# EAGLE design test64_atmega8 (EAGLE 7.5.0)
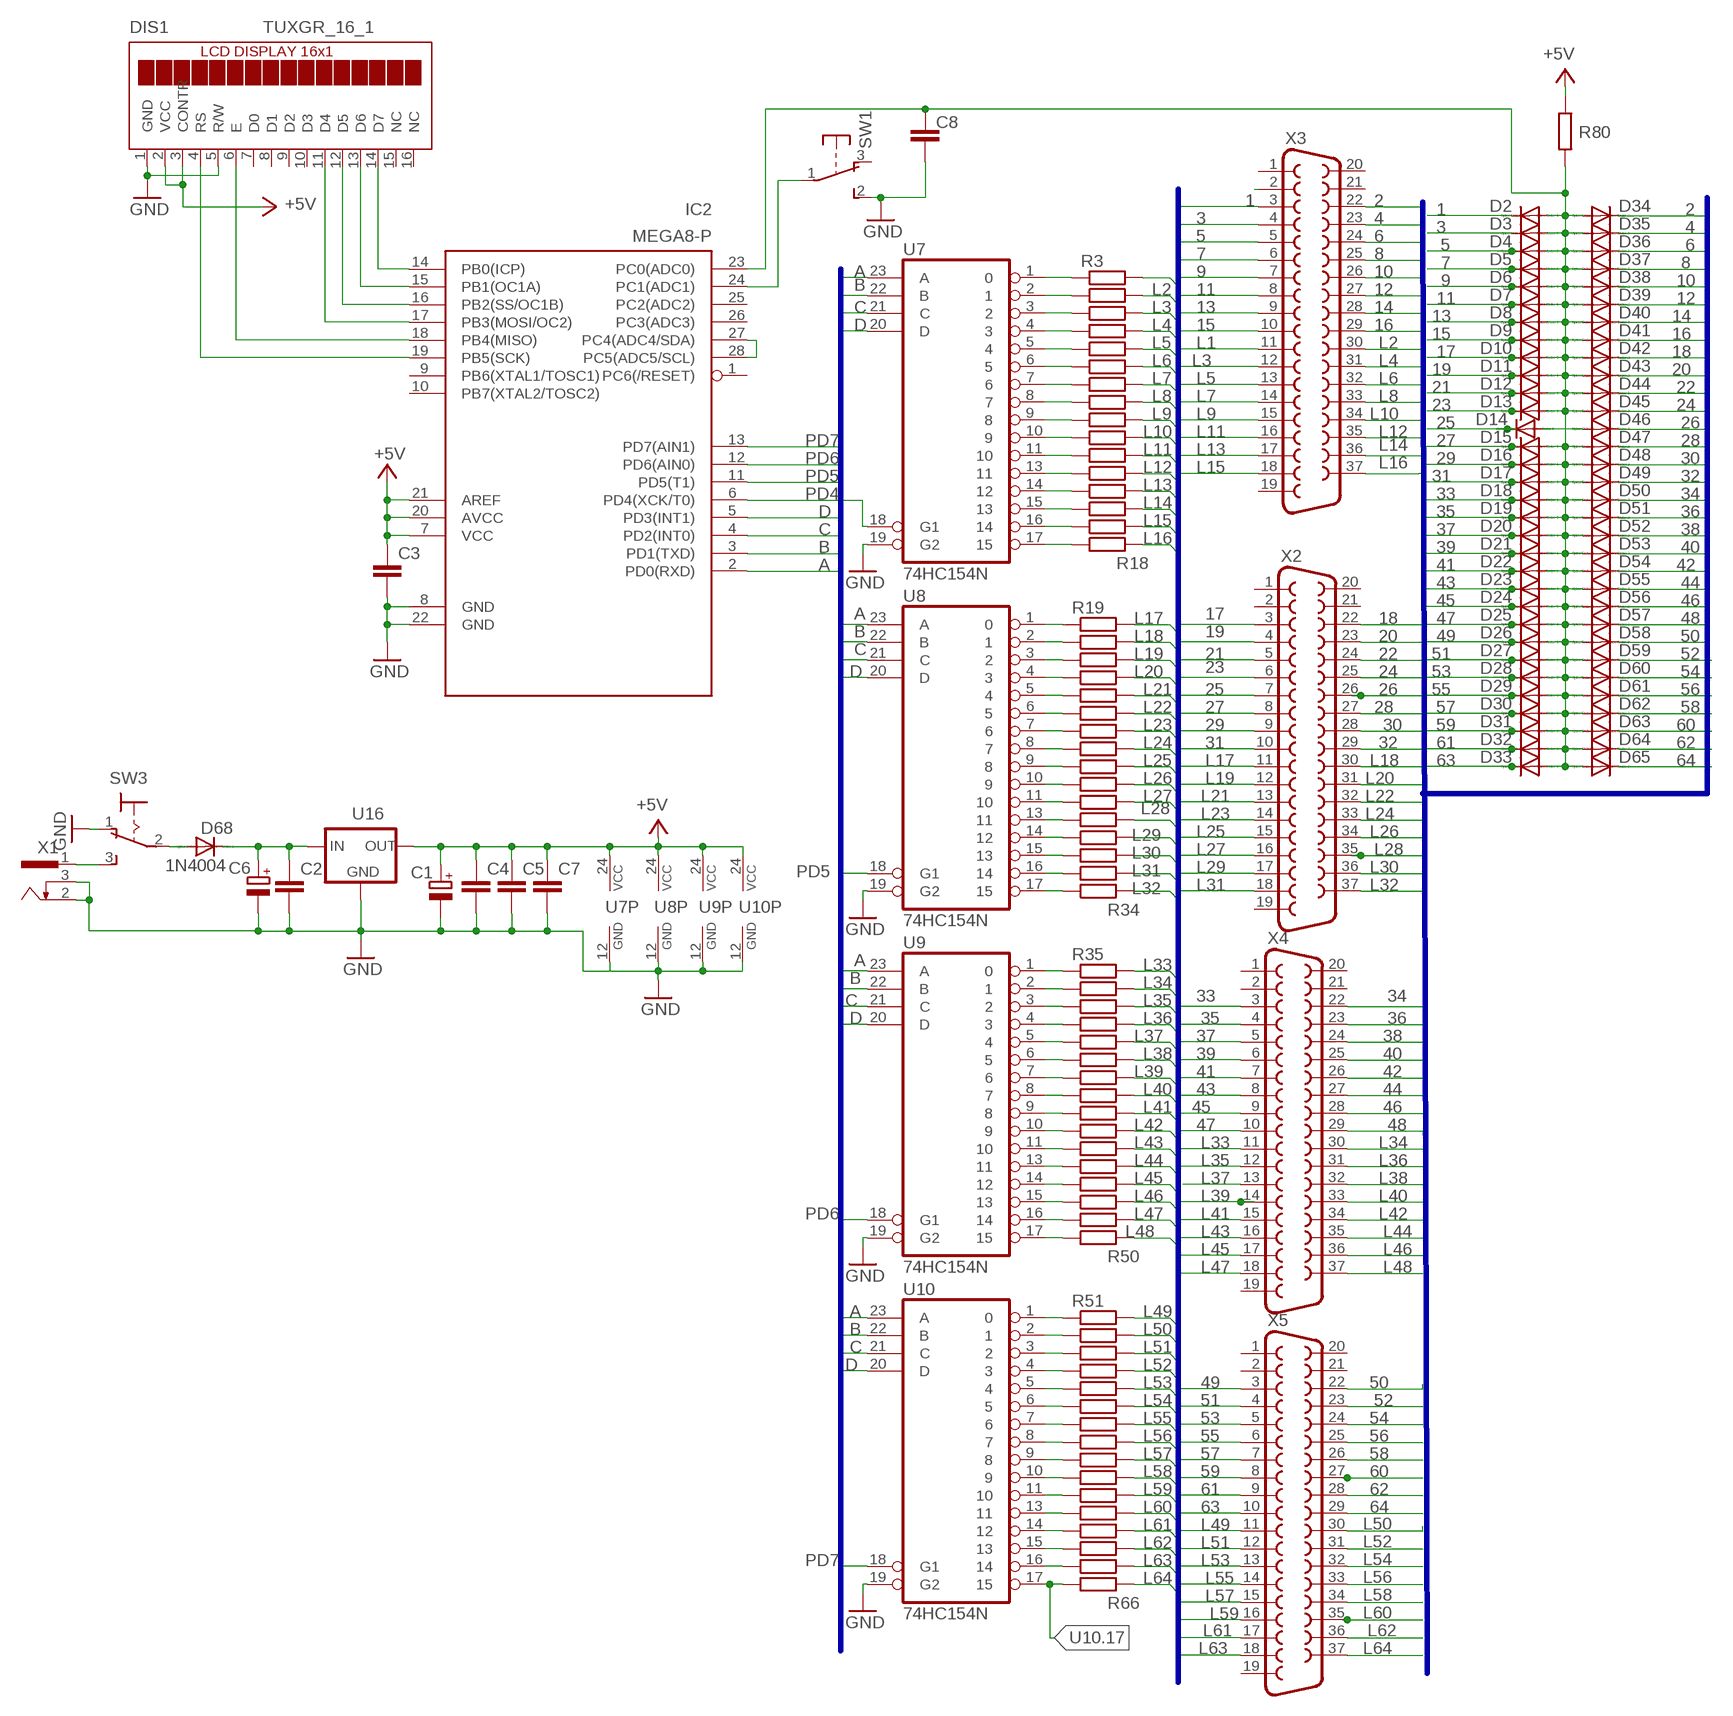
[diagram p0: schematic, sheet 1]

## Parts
C1  CPOL-EUC/6032-28W  [C/6032-28W]
C2  C-EUC1206  [C1206]
C3  C-EUC1206  [C1206]
C4  C-EUC1206  [C1206]
C5  C-EUC1206  [C1206]
C6  CPOL-EUC/6032-28W  [C/6032-28W]
C7  C-EUC1206  [C1206]
C8  C-EUC1206  [C1206]
D2  1N4148DO35-7  [DO35-7]
D3  1N4148DO35-7  [DO35-7]
D4  1N4148DO35-7  [DO35-7]
D5  1N4148DO35-7  [DO35-7]
D6  1N4148DO35-7  [DO35-7]
D7  1N4148DO35-7  [DO35-7]
D8  1N4148DO35-7  [DO35-7]
D9  1N4148DO35-7  [DO35-7]
D10  1N4148DO35-7  [DO35-7]
D11  1N4148DO35-7  [DO35-7]
D12  1N4148DO35-7  [DO35-7]
D13  1N4148DO35-7  [DO35-7]
D14  1N4148DO35-7  [DO35-7]
D15  1N4148DO35-7  [DO35-7]
D16  1N4148DO35-7  [DO35-7]
D17  1N4148DO35-7  [DO35-7]
D18  1N4148DO35-7  [DO35-7]
D19  1N4148DO35-7  [DO35-7]
D20  1N4148DO35-7  [DO35-7]
D21  1N4148DO35-7  [DO35-7]
D22  1N4148DO35-7  [DO35-7]
D23  1N4148DO35-7  [DO35-7]
D24  1N4148DO35-7  [DO35-7]
D25  1N4148DO35-7  [DO35-7]
D26  1N4148DO35-7  [DO35-7]
D27  1N4148DO35-7  [DO35-7]
D28  1N4148DO35-7  [DO35-7]
D29  1N4148DO35-7  [DO35-7]
D30  1N4148DO35-7  [DO35-7]
D31  1N4148DO35-7  [DO35-7]
D32  1N4148DO35-7  [DO35-7]
D33  1N4148DO35-7  [DO35-7]
D34  1N4148DO35-7  [DO35-7]
D35  1N4148DO35-7  [DO35-7]
D36  1N4148DO35-7  [DO35-7]
D37  1N4148DO35-7  [DO35-7]
D38  1N4148DO35-7  [DO35-7]
D39  1N4148DO35-7  [DO35-7]
D40  1N4148DO35-7  [DO35-7]
D41  1N4148DO35-7  [DO35-7]
D42  1N4148DO35-7  [DO35-7]
D43  1N4148DO35-7  [DO35-7]
D44  1N4148DO35-7  [DO35-7]
D45  1N4148DO35-7  [DO35-7]
D46  1N4148DO35-7  [DO35-7]
D47  1N4148DO35-7  [DO35-7]
D48  1N4148DO35-7  [DO35-7]
D49  1N4148DO35-7  [DO35-7]
D50  1N4148DO35-7  [DO35-7]
D51  1N4148DO35-7  [DO35-7]
D52  1N4148DO35-7  [DO35-7]
D53  1N4148DO35-7  [DO35-7]
D54  1N4148DO35-7  [DO35-7]
D55  1N4148DO35-7  [DO35-7]
D56  1N4148DO35-7  [DO35-7]
D57  1N4148DO35-7  [DO35-7]
D58  1N4148DO35-7  [DO35-7]
D59  1N4148DO35-7  [DO35-7]
D60  1N4148DO35-7  [DO35-7]
D61  1N4148DO35-7  [DO35-7]
D62  1N4148DO35-7  [DO35-7]
D63  1N4148DO35-7  [DO35-7]
D64  1N4148DO35-7  [DO35-7]
D65  1N4148DO35-7  [DO35-7]
D68  1N4004  [DO41-10]
DIS1  TUXGR_16_1  [TUXGR_16X1]
IC2  MEGA8-P  [DIL28-3]
R3  R-EU_R1206  [R1206]
R4  R-EU_R1206  [R1206]
R5  R-EU_R1206  [R1206]
R6  R-EU_R1206  [R1206]
R7  R-EU_R1206  [R1206]
R8  R-EU_R1206  [R1206]
R9  R-EU_R1206  [R1206]
R10  R-EU_R1206  [R1206]
R11  R-EU_R1206  [R1206]
R12  R-EU_R1206  [R1206]
R13  R-EU_R1206  [R1206]
R14  R-EU_R1206  [R1206]
R15  R-EU_R1206  [R1206]
R16  R-EU_R1206  [R1206]
R17  R-EU_R1206  [R1206]
R18  R-EU_R1206  [R1206]
R19  R-EU_R1206  [R1206]
R20  R-EU_R1206  [R1206]
R21  R-EU_R1206  [R1206]
R22  R-EU_R1206  [R1206]
R23  R-EU_R1206  [R1206]
R24  R-EU_R1206  [R1206]
R25  R-EU_R1206  [R1206]
R26  R-EU_R1206  [R1206]
R27  R-EU_R1206  [R1206]
R28  R-EU_R1206  [R1206]
R29  R-EU_R1206  [R1206]
R30  R-EU_R1206  [R1206]
R31  R-EU_R1206  [R1206]
R32  R-EU_R1206  [R1206]
R33  R-EU_R1206  [R1206]
R34  R-EU_R1206  [R1206]
R35  R-EU_R1206  [R1206]
R36  R-EU_R1206  [R1206]
R37  R-EU_R1206  [R1206]
R38  R-EU_R1206  [R1206]
R39  R-EU_R1206  [R1206]
R40  R-EU_R1206  [R1206]
R41  R-EU_R1206  [R1206]
R42  R-EU_R1206  [R1206]
R43  R-EU_R1206  [R1206]
R44  R-EU_R1206  [R1206]
R45  R-EU_R1206  [R1206]
R46  R-EU_R1206  [R1206]
R47  R-EU_R1206  [R1206]
R48  R-EU_R1206  [R1206]
R49  R-EU_R1206  [R1206]
R50  R-EU_R1206  [R1206]
R51  R-EU_R1206  [R1206]
R52  R-EU_R1206  [R1206]
R53  R-EU_R1206  [R1206]
R54  R-EU_R1206  [R1206]
R55  R-EU_R1206  [R1206]
R56  R-EU_R1206  [R1206]
R57  R-EU_R1206  [R1206]
R58  R-EU_R1206  [R1206]
R59  R-EU_R1206  [R1206]
R60  R-EU_R1206  [R1206]
R61  R-EU_R1206  [R1206]
R62  R-EU_R1206  [R1206]
R63  R-EU_R1206  [R1206]
R64  R-EU_R1206  [R1206]
R65  R-EU_R1206  [R1206]
R66  R-EU_R1206  [R1206]
R80  R-EU_R1206  [R1206]
SW1  9077-1  [9077-1]
SW3  320-916  [320-916]
U7  74HC154N  [DIL24-6]
U8  74HC154N  [DIL24-6]
U9  74HC154N  [DIL24-6]
U10  74HC154N  [DIL24-6]
U16  78XXL  [78XXL]
X1  733980-62  [733980-62]
X2  F37V  [F37V]
X3  F37V  [F37V]
X4  F37V  [F37V]
X5  F37V  [F37V]

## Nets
1: D2.C X3.3
2: D34.C X3.22
3: D3.C X3.4
4: D35.C X3.23
5: D4.C X3.5
6: D36.C X3.24
7: D5.C X3.6
8: D37.C X3.25
9: D6.C X3.7
10: D38.C X3.26
11: D7.C X3.8
12: D39.C X3.27
13: D8.C X3.9
14: D40.C X3.28
15: D9.C X3.10
16: D41.C X3.29
17: D10.C X2.3
18: D42.C X2.22
19: D11.C X2.4
20: D43.C X2.23
21: D12.C X2.5
22: D44.C X2.24
23: D13.C X2.6
24: D45.C X2.25
25: D14.C X2.7
26: D46.C X2.26
27: D15.C X2.8
28: D47.C X2.27
29: D16.C X2.9
30: D48.C X2.28
31: D17.C X2.10
32: D49.C X2.29
33: D18.C X4.3
34: D50.C X4.22
35: D19.C X4.4
36: D51.C X4.23
37: D20.C X4.5
38: D52.C X4.24
39: D21.C X4.6
40: D53.C X4.25
41: D22.C X4.7
42: D54.C X4.26
43: D23.C X4.8
44: D55.C X4.27
45: D24.C X4.9
46: D56.C X4.28
47: D25.C X4.10
48: D57.C X4.29
49: D26.C X5.3
50: D58.C X5.22
51: D27.C X5.4
52: D59.C X5.23
53: D28.C X5.5
54: D60.C X5.24
55: D29.C X5.6
56: D61.C X5.25
57: D30.C X5.7
58: D62.C X5.26
59: D31.C X5.8
60: D63.C X5.27
61: D32.C X5.9
62: D64.C X5.28
63: D33.C X5.10
64: D65.C X5.29
+5V: C1.+ C3.1 C4.1 C5.1 C7.1 DIS1.2(VCC) DIS1.3(CONTR) IC2.7(VCC) IC2.20(AVCC) IC2.21(AREF) R80.1 U7.24(VCC) U8.24(VCC) U9.24(VCC) U10.24(VCC) U16.OUT
A: IC2.2(PD0(RXD)) U7.23(A) U8.23(A) U9.23(A) U10.23(A)
B: IC2.3(PD1(TXD)) U7.22(B) U8.22(B) U9.22(B) U10.22(B)
C: IC2.4(PD2(INT0)) U7.21(C) U8.21(C) U9.21(C) U10.21(C)
D: IC2.5(PD3(INT1)) U7.20(D) U8.20(D) U9.20(D) U10.20(D)
GND: C1.- C2.2 C3.2 C4.2 C5.2 C6.- C7.2 C8.2 DIS1.1(GND) DIS1.5(R/W) IC2.8(GND) IC2.22(GND) SW1.2(S) SW3.1(O) U7.12(GND) U7.19(G2) U8.12(GND) U8.19(G2) U9.12(GND) U9.19(G2) U10.12(GND) U10.19(G2) U16.GND X1.2 X1.3
L1: R3.2 X3.11
L2: R4.2 X3.30
L3: R5.2 X3.12
L4: R6.2 X3.31
L5: R7.2 X3.13
L6: R8.2 X3.32
L7: R9.2 X3.14
L8: R10.2 X3.33
L9: R11.2 X3.15
L10: R12.2 X3.34
L11: R13.2 X3.16
L12: R14.2 X3.35
L13: R15.2 X3.17
L14: R16.2 X3.36
L15: R17.2 X3.18
L16: R18.2 X3.37
L17: R19.2 X2.11
L18: R20.2 X2.30
L19: R21.2 X2.12
L20: R22.2 X2.31
L21: R23.2 X2.13
L22: R24.2 X2.32
L23: R25.2 X2.14
L24: R26.2 X2.33
L25: R27.2 X2.15
L26: R28.2 X2.34
L27: R29.2 X2.16
L28: R30.2 X2.35
L29: R31.2 X2.17
L30: R32.2 X2.36
L31: R33.2 X2.18
L32: R34.2 X2.37
L33: R35.2 X4.11
L34: R36.2 X4.30
L35: R37.2 X4.12
L36: R38.2 X4.31
L37: R39.2 X4.13
L38: R40.2 X4.32
L39: R41.2 X4.14
L40: R42.2 X4.33
L41: R43.2 X4.15
L42: R44.2 X4.34
L43: R45.2 X4.16
L44: R46.2 X4.35
L45: R47.2 X4.17
L46: R48.2 X4.36
L47: R49.2 X4.18
L48: R50.2 X4.37
L49: R51.2 X5.11
L50: R52.2 X5.30
L51: R53.2 X5.12
L52: R54.2 X5.31
L53: R55.2 X5.13
L54: R56.2 X5.32
L55: R57.2 X5.14
L56: R58.2 X5.33
L57: R59.2 X5.15
L58: R60.2 X5.34
L59: R61.2 X5.16
L60: R62.2 X5.35
L61: R63.2 X5.17
L62: R64.2 X5.36
L63: R65.2 X5.18
L64: R66.2 X5.37
N$1: IC2.27(PC4(ADC4/SDA)) IC2.28(PC5(ADC5/SCL))
N$2: IC2.24(PC1(ADC1)) SW1.1(P)
N$3: DIS1.14(D7) IC2.14(PB0(ICP))
N$4: DIS1.13(D6) IC2.15(PB1(OC1A))
N$5: DIS1.12(D5) IC2.16(PB2(SS/OC1B))
N$6: DIS1.11(D4) IC2.17(PB3(MOSI/OC2))
N$7: R4.1 U7.2
N$8: R5.1 U7.3
N$9: R6.1 U7.4
N$10: R7.1 U7.5
N$11: R8.1 U7.6
N$12: R9.1 U7.7
N$13: R10.1 U7.8
N$14: R11.1 U7.9
N$15: R12.1 U7.10
N$16: R13.1 U7.11
N$17: R14.1 U7.13
N$18: R15.1 U7.14
N$19: R16.1 U7.15
N$20: R17.1 U7.16
N$21: R18.1 U7.17
N$22: R19.1 U8.1
N$23: R20.1 U8.2
N$24: R21.1 U8.3
N$25: R22.1 U8.4
N$26: R23.1 U8.5
N$27: R24.1 U8.6
N$28: R25.1 U8.7
N$29: R26.1 U8.8
N$30: R27.1 U8.9
N$31: R28.1 U8.10
N$32: R29.1 U8.11
N$33: R30.1 U8.13
N$34: R31.1 U8.14
N$35: R32.1 U8.15
N$36: R33.1 U8.16
N$37: R34.1 U8.17
N$38: R35.1 U9.1
N$39: R36.1 U9.2
N$40: R37.1 U9.3
N$41: R38.1 U9.4
N$42: R39.1 U9.5
N$43: R40.1 U9.6
N$44: R41.1 U9.7
N$45: R42.1 U9.8
N$46: R43.1 U9.9
N$47: R44.1 U9.10
N$48: R45.1 U9.11
N$49: R46.1 U9.13
N$50: R47.1 U9.14
N$51: R48.1 U9.15
N$52: R49.1 U9.16
N$53: R50.1 U9.17
N$54: R51.1 U10.1
N$55: R52.1 U10.2
N$56: R53.1 U10.3
N$57: R54.1 U10.4
N$58: R55.1 U10.5
N$59: R56.1 U10.6
N$60: R57.1 U10.7
N$61: R58.1 U10.8
N$62: R59.1 U10.9
N$63: R60.1 U10.10
N$64: R61.1 U10.11
N$65: R62.1 U10.13
N$66: R63.1 U10.14
N$67: R64.1 U10.15
N$68: R65.1 U10.16
N$69: DIS1.6(E) IC2.18(PB4(MISO))
N$70: DIS1.4(RS) IC2.19(PB5(SCK))
N$71: X3.2
N$72: R3.1 U7.1
N$95: D68.A SW3.2(P)
N$109: C8.1 D2.A D3.A D4.A D5.A D6.A D7.A D8.A D9.A D10.A D11.A D12.A D13.A D14.A D15.A D16.A D17.A D18.A D19.A D20.A D21.A D22.A D23.A D24.A D25.A D26.A D27.A D28.A D29.A D30.A D31.A D32.A D33.A D34.A D35.A D36.A D37.A D38.A D39.A D40.A D41.A D42.A D43.A D44.A D45.A D46.A D47.A D48.A D49.A D50.A D51.A D52.A D53.A D54.A D55.A D56.A D57.A D58.A D59.A D60.A D61.A D62.A D63.A D64.A D65.A IC2.23(PC0(ADC0)) R80.2
N$118: C2.1 C6.+ D68.C U16.IN
N$119: SW3.3(S) X1.1
PD4: IC2.6(PD4(XCK/T0)) U7.18(G1)
PD5: IC2.11(PD5(T1)) U8.18(G1)
PD6: IC2.12(PD6(AIN0)) U9.18(G1)
PD7: IC2.13(PD7(AIN1)) U10.18(G1)
U10.17: R66.1 U10.17
Unconnected: DIS1.7(D0) DIS1.8(D1) DIS1.9(D2) DIS1.10(D3) DIS1.15(NC) DIS1.16(NC) IC2.1(PC6(/RESET)) IC2.9(PB6(XTAL1/TOSC1)) IC2.10(PB7(XTAL2/TOSC2)) IC2.25(PC2(ADC2)) IC2.26(PC3(ADC3)) SW1.3(O) X2.1 X2.2 X2.19 X2.20 X2.21 X3.1 X3.19 X3.20 X3.21 X4.1 X4.2 X4.19 X4.20 X4.21 X5.1 X5.2 X5.19 X5.20 X5.21

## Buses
B$1
B$2
B$3

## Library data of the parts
C1 C6 = rcl:CPOL-EU: POLARIZED CAPACITOR, European symbol
C2-C5 C7 C8 = rcl:C-EU: CAPACITOR, European symbol
D2-D65 = diode:1N4148: DIODE
D68 = diode:1N4004: DIODE
DIS1 = display-lcd:TUXGR_16_1: 1x16 LCD DISPLAY
IC2 = atmel:MEGA8-P: MICROCONTROLLER 8 Kbytes FLASH, 1 kbytes SRAM, 512 bytes EEPROM, USART, 4-channel 10 bit ADC, 2-channel 8 bit ADC Pin compatible with Atmega48, ATMega88, ATMega168 Source: avr.lbr; OC_FARNELL: unknown; OC_NEWARK: unknown
R3-R66 R80 = rcl:R-EU_: RESISTOR, European symbol
SW1 = switch-misc:9077-1: MARQUARDT SWITCH 9077.0100 Distributor: Buerklin
SW3 = switch:320-916: TOGGLE SWITCH distributor RS Components
U7-U10 = 74xx-eu:74*154: 4-line to 16-line data SELECTOR/MULTIPLEXER
U16 = v-reg:78XXL: VOLTAGE REGULATOR
X1 = con-conrad:73398?: FEMALE PRINT CONNECTOR Niedervolt-Steckverbinder Distributor Conrad
X2-X5 = con-subd:F37: SUB-D; OC_FARNELL: unknown; OC_NEWARK: unknown

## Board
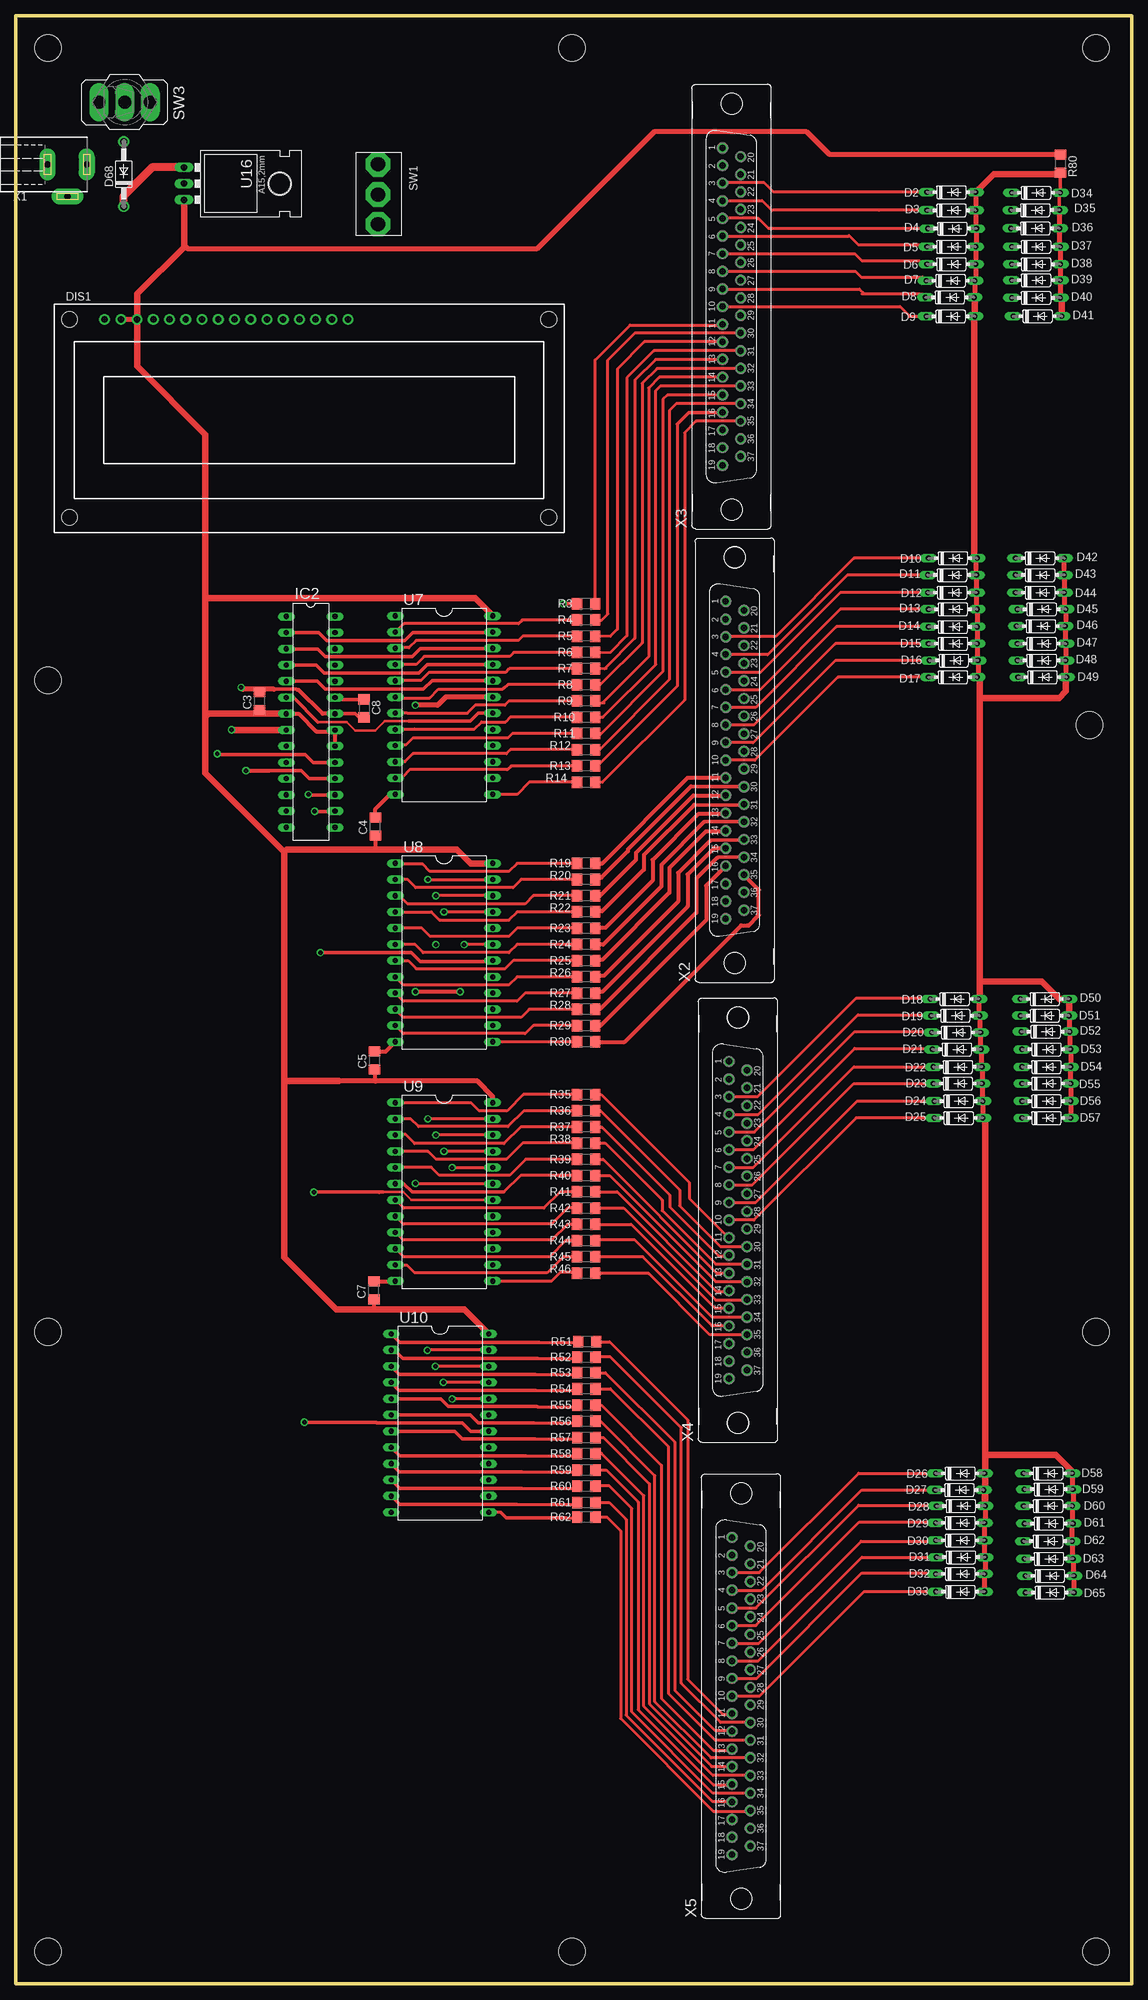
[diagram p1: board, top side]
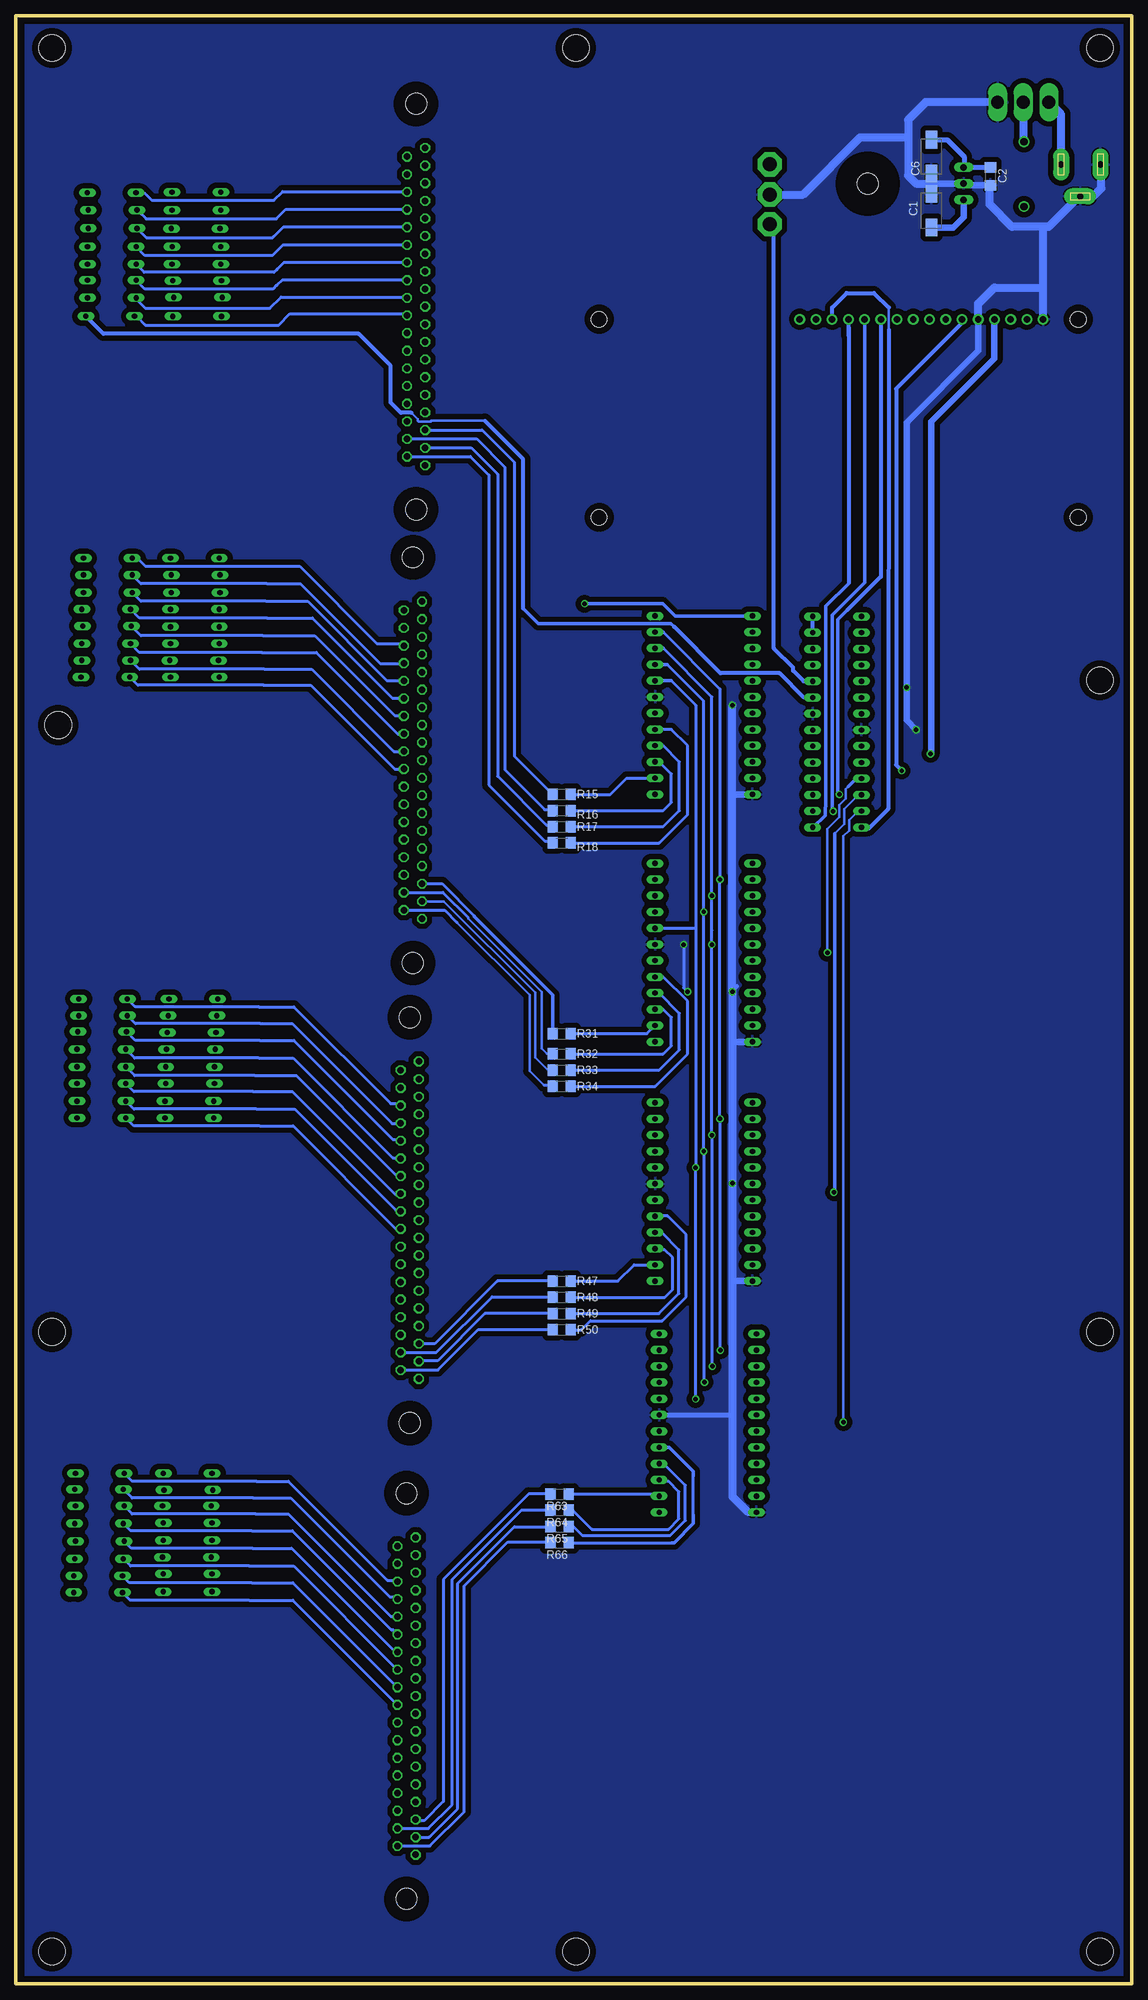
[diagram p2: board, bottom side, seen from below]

Size 174.62 x 308 mm. Coordinates in mm from the lower left corner, seen from the top.
Outline: 0,0 0,308 174.62,308 174.62,0 0,0
Copper layers (1*16): Top 0.035mm / dielectric 1.5mm / Bottom 0.035mm
Design rules "default *": minimum track width 10mil, minimum drill 24mil, track to track 8mil, track to pad 8mil, pad to pad 8mil, via to via 8mil, smd to smd 8mil, copper to edge 40mil, drill to drill 8mil, minimum pad ring 10mil, minimum via ring 8mil, stop-mask expansion 4mil, vias tented up to drill 0mil, thermal gap 10mil
Holes 4.2 mm at 5,303 5,5 5,204 5,102 169,5 169,102 168,197 169,303 87,303 87,5

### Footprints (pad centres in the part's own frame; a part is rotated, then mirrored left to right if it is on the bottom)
C/6032-28W = smd 2.75 x 1.8: + 2.625,0; - -2.625,0
C1206 = smd 1.6 x 1.8: 1 -1.4,0; 2 1.4,0
DO35-7 = drill 0.813 long: A 3.81,0; C -3.81,0
DO41-10 = drill 1.118: A 5.08,0; C -5.08,0
TUXGR_16X1 = drill 1 pad 1.676: 1 -0.25,0.26; 2 2.29,0.26; 3 4.83,0.26; 4 7.37,0.26; 5 9.91,0.26; 6 12.45,0.26; 7 14.99,0.26; 8 17.53,0.26; 9 20.07,0.26; 10 22.61,0.26; 11 25.15,0.26; 12 27.69,0.26; 13 30.23,0.26; 14 32.77,0.26; 15 35.31,0.26; 16 37.85,0.26 | hole 2.5: -5.75,-30.74; 69.25,-30.74; -5.75,0.26; 69.25,0.26
DIL28-3 = drill 0.813 long: 1 -16.51,-3.81; 2 -13.97,-3.81; 3 -11.43,-3.81; 4 -8.89,-3.81; 5 -6.35,-3.81; 6 -3.81,-3.81; 7 -1.27,-3.81; 8 1.27,-3.81; 9 3.81,-3.81; 10 6.35,-3.81; 11 8.89,-3.81; 12 11.43,-3.81; 13 13.97,-3.81; 14 16.51,-3.81; 15 16.51,3.81; 16 13.97,3.81; 17 11.43,3.81; 18 8.89,3.81; 19 6.35,3.81; 20 3.81,3.81; 21 1.27,3.81; 22 -1.27,3.81; 23 -3.81,3.81; 24 -6.35,3.81; 25 -8.89,3.81; 26 -11.43,3.81; 27 -13.97,3.81; 28 -16.51,3.81
R1206 = smd 1.6 x 1.803: 1 -1.422,0; 2 1.422,0
9077-1 = drill 2.2 pad 3.81 octagon: 1 4.7,-0.116; 2 0.06,-0.116; 3 -4.66,-0.116
320-916 = drill 2.007 long: 1 0,4.013; 2 0,0; 3 0,-4.013
DIL24-6 = drill 0.813 long: 1 -13.97,-7.62; 2 -11.43,-7.62; 3 -8.89,-7.62; 4 -6.35,-7.62; 5 -3.81,-7.62; 6 -1.27,-7.62; 7 1.27,-7.62; 8 3.81,-7.62; 9 6.35,-7.62; 10 8.89,-7.62; 11 11.43,-7.62; 12 13.97,-7.62; 13 13.97,7.62; 14 11.43,7.62; 15 8.89,7.62; 16 6.35,7.62; 17 3.81,7.62; 18 1.27,7.62; 19 -1.27,7.62; 20 -3.81,7.62; 21 -6.35,7.62; 22 -8.89,7.62; 23 -11.43,7.62; 24 -13.97,7.62
78XXL = drill 1.016 long: GND 0,-3.81; IN -2.54,-3.81; OUT 2.54,-3.81 | hole 3.302: 0,11.176
733980-62 = drill 1 pad 2.5 long: 1 0,8.57; 2 0,2.42; 3 5,5.57
F37V = drill 1.016 octagon: 1 24.841,1.422; 2 22.073,1.422; 3 19.329,1.422; 4 16.561,1.422; 5 13.792,1.422; 6 11.049,1.422; 7 8.28,1.422; 8 5.512,1.422; 9 2.769,1.422; 10 0,1.422; 11 -2.769,1.422; 12 -5.512,1.422; 13 -8.28,1.422; 14 -11.049,1.422; 15 -13.818,1.422; 16 -16.561,1.422; 17 -19.329,1.422; 18 -22.098,1.422; 19 -24.841,1.422; 20 23.47,-1.422; 21 20.701,-1.422; 22 17.932,-1.422; 23 15.189,-1.422; 24 12.421,-1.422; 25 9.652,-1.422; 26 6.909,-1.422; 27 4.14,-1.422; 28 1.372,-1.422; 29 -1.372,-1.422; 30 -4.14,-1.422; 31 -6.909,-1.422; 32 -9.677,-1.422; 33 -12.421,-1.422; 34 -15.189,-1.422; 35 -17.958,-1.422; 36 -20.701,-1.422; 37 -23.47,-1.422 | hole 3.302: 31.75,0; -31.75,0

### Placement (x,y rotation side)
C1  31.38,277.5 270 bottom
C2  22.12,282.88 270 bottom
C3  38.12,200.75 90 top
C4  56.25,181.12 90 top
C5  56.12,144.5 90 top
C6  31.38,286 90 bottom
C7  56,108.5 90 top
C8  54.5,199.62 270 top
D2  146.38,280.43 0 top
D3  146.38,277.57 0 top
D4  146.51,274.73 0 top
D5  146.38,271.88 0 top
D6  146.38,269.15 0 top
D7  146.26,266.55 0 top
D8  146.13,263.95 0 top
D9  146.26,260.98 0 top
D10  146.62,223.12 0 top
D11  146.5,220.5 0 top
D12  146.5,217.75 0 top
D13  146.62,215.12 0 top
D14  146.62,212.38 0 top
D15  146.62,209.75 0 top
D16  146.75,207.12 0 top
D17  146.62,204.5 0 top
D18  146.88,154.12 0 top
D19  147,151.5 0 top
D20  147.12,148.88 0 top
D21  147.25,146.25 0 top
D22  147.38,143.5 0 top
D23  147.38,140.88 0 top
D24  147.5,138.12 0 top
D25  147.5,135.5 0 top
D26  147.75,79.88 0 top
D27  147.64,77.25 0 top
D28  147.88,74.75 0 top
D29  147.75,72.12 0 top
D30  147.75,69.38 0 top
D31  147.88,66.75 0 top
D32  147.75,64.12 0 top
D33  147.76,61.35 0 top
D34  159.64,280.32 0 top
D35  159.5,277.62 0 top
D36  159.5,274.75 0 top
D37  159.62,271.88 0 top
D38  159.62,269.12 0 top
D39  159.62,266.62 0 top
D40  159.62,263.88 0 top
D41  159.88,261 0 top
D42  160.25,223.12 0 top
D43  160.25,220.5 0 top
D44  160.25,217.75 0 top
D45  160.5,215.12 0 top
D46  160.38,212.5 0 top
D47  160.5,209.75 0 top
D48  160.5,207.12 0 top
D49  160.62,204.5 0 top
D50  161,154.12 0 top
D51  161,151.5 0 top
D52  161.12,149 0 top
D53  161.25,146.25 0 top
D54  161.25,143.5 0 top
D55  161.25,140.88 0 top
D56  161.25,138.12 0 top
D57  161.25,135.5 0 top
D58  161.5,79.88 0 top
D59  161.62,77.38 0 top
D60  161.5,74.75 0 top
D61  161.62,72 0 top
D62  161.5,69.25 0 top
D63  161.62,66.5 0 top
D64  161.76,63.83 0 top
D65  161.78,61.2 0 top
D68  16.88,283.25 90 top
DIS1  14.12,260.25 0 top
IC2  46.12,197.5 270 top
R3  89.22,216 0 top
R4  89.22,213.46 0 top
R5  89.22,210.92 0 top
R6  89.22,208.38 0 top
R7  89.22,205.84 0 top
R8  89.22,203.3 0 top
R9  89.22,200.76 0 top
R10  89.22,198.22 0 top
R11  89.22,195.68 0 top
R12  89.22,193.14 0 top
R13  89.22,190.6 0 top
R14  89.22,188.06 0 top
R15  89.22,186.16 180 bottom
R16  89.22,183.62 180 bottom
R17  89.22,181.07 180 bottom
R18  89.22,178.53 180 bottom
R19  89.22,175.36 0 top
R20  89.22,172.82 0 top
R21  89.22,170.28 0 top
R22  89.22,167.74 0 top
R23  89.22,165.2 0 top
R24  89.22,162.66 0 top
R25  89.22,160.12 0 top
R26  89.22,157.58 0 top
R27  89.22,155.04 0 top
R28  89.22,152.5 0 top
R29  89.22,149.96 0 top
R30  89.22,147.42 0 top
R31  89.22,148.69 180 bottom
R32  89.22,145.51 180 bottom
R33  89.22,142.97 180 bottom
R34  89.22,140.44 180 bottom
R35  89.22,139.16 0 top
R36  89.22,136.62 0 top
R37  89.22,134.09 0 top
R38  89.22,131.54 0 top
R39  89.22,129 0 top
R40  89.22,126.47 0 top
R41  89.22,123.92 0 top
R42  89.22,121.39 0 top
R43  89.22,118.84 0 top
R44  89.22,116.31 0 top
R45  89.22,113.77 0 top
R46  89.22,111.22 0 top
R47  89.22,109.95 180 bottom
R48  89.22,107.42 180 bottom
R49  89.22,104.88 180 bottom
R50  89.22,102.33 180 bottom
R51  89.41,100.45 0 top
R52  89.28,98.04 0 top
R53  89.28,95.62 0 top
R54  89.28,93.08 0 top
R55  89.28,90.54 0 top
R56  89.28,88 0 top
R57  89.28,85.46 0 top
R58  89.28,82.92 0 top
R59  89.28,80.38 0 top
R60  89.28,77.84 0 top
R61  89.28,75.3 0 top
R62  89.28,73.01 0 top
R63  89.53,76.62 180 bottom
R64  89.53,74.08 180 bottom
R65  89.53,71.54 180 bottom
R66  89.53,69 180 bottom
R80  163.5,284.88 270 top
SW1  56.77,280.11 270 top
SW3  17,294.5 270 top
U7  66.99,200.12 270 top
U8  66.99,161.39 270 top
U9  66.99,123.92 270 top
U10  66.36,87.73 270 top
U16  30.12,281.75 270 top
X1  2.5,284.75 270 top
X2  112.5,191.5 90 top
X3  112,262.5 90 top
X4  113,119.5 90 top
X5  113.5,45 90 top

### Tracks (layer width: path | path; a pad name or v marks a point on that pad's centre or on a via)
1
  Top 0.5: 133.1,280.43 118.58,280.43 117.12,281.88 110.62,281.88 X3.3
  Top 0.506: D2.C 133.1,280.43
2
  Bottom 0.5: 134.34,279.12 134.25,279.12 132.88,280.5 113.49,280.5 X3.22
  Bottom 0.506: D34.C 154.57,280.32 153.38,279.12 134.34,279.12
3
  Top 0.5: 135.07,277.57 118.3,277.57 116.75,279.12 116.69,279.06 X3.4
  Top 0.506: D3.C 135.07,277.57
4
  Bottom 0.5: 134,276.25 133.88,276.25 132.38,277.75 113.48,277.75 X3.23
  Bottom 0.506: D35.C 155.62,277.62 154.25,276.25 134,276.25
5
  Top 0.5: 132.48,274.73 117.78,274.73 116.25,276.25 116.12,276.25 116,276.38 110.66,276.38 X3.5
  Top 0.506: D4.C 132.48,274.73
6
  Bottom 0.5: 134.29,273.45 132.75,275 113.5,275 X3.24
  Bottom 0.506: 134.29,273.45 134.5,273.25 154.19,273.25 D36.C
7
  Top 0.5: 132.42,272.12 131.88,272.12 130.38,273.62 130.3,273.55 X3.6
  Top 0.506: D5.C 141.62,271.88 141.38,272.12 132.42,272.12
8
  Bottom 0.5: X3.25 132.85,272.15 134.09,270.92
  Bottom 0.506: 134.09,270.92 134.5,270.5 154.44,270.5 D37.C
9
  Top 0.5: X3.7 131.3,270.78 132.46,269.62
  Top 0.506: D6.C 141.85,269.15 141.38,269.62 132.46,269.62
10
  Bottom 0.5: X3.26 132.72,269.41 133.75,268.38
  Bottom 0.506: 133.75,268.38 134.25,267.88 154.56,267.88 D38.C
11
  Top 0.5: X3.8 131.36,268.01 132.25,267.12
  Top 0.506: 132.25,267.12 141.87,267.12 D7.C
12
  Bottom 0.5: X3.27 132.99,266.64 133.79,265.83
  Bottom 0.506: 133.79,265.83 134.38,265.25 154.44,265.25 D39.C
13
  Top 0.5: X3.9 131.98,265.27 132.75,264.5
  Top 0.506: 132.38,264.5 132.75,264.5 141.77,264.5 D8.C
14
  Bottom 0.5: D40.C 155.81,263.69 154.38,262.25 134.88,262.25 133.12,264 113.55,264 X3.28
15
  Top 0.5: X3.10 138.38,262.5 139.88,261 142.42,261 D9.C
16
  Bottom 0.5: D41.C 155.75,261 154.38,259.62 133.5,259.62 131.75,261.38 113.67,261.38 X3.29
17
  Top 0.5: D10.C 131.12,223.12 118.88,210.88 111.12,210.88 X2.3
18
  Bottom 0.5: D42.C 155.62,223.12 154.38,221.88 130.25,221.88 118.12,209.75 114.24,209.75 X2.22
19
  Top 0.5: D11.C 130.12,220.5 117.62,208 111.14,208 X2.4
20
  Bottom 0.5: 135.38,219.12 130.12,219.12 117.62,206.62 113.99,206.62 X2.23
  Bottom 0.506: 135.38,219.12 155.06,219.12 D43.C
21
  Top 0.5: D12.C 129,217.75 116.5,205.25 111.12,205.25 X2.5
22
  Bottom 0.5: 135.5,216.38 129,216.38 116.62,204 114,204 X2.24
  Bottom 0.506: 135.5,216.38 155.06,216.38 D44.C
23
  Top 0.5: D13.C 129,215.12 116.38,202.5 111.13,202.5 X2.6
24
  Bottom 0.5: 135.38,213.75 128.25,213.75 115.75,201.25 114.02,201.25 X2.25
  Bottom 0.506: 135.38,213.75 155.31,213.75 D45.C
25
  Top 0.5: D14.C 128.38,212.38 115.75,199.75 111.11,199.75 X2.7
26
  Bottom 0.5: 136,211 127.88,211 115.38,198.5 114.01,198.5 X2.26
  Bottom 0.506: 136,211 155.06,211 D46.C
27
  Top 0.5: D15.C 128.25,209.75 115.5,197 X2.8
28
  Bottom 0.5: 136.12,208.38 127.62,208.38 114.88,195.62 113.94,195.62 X2.27
  Bottom 0.506: 136.12,208.38 155.31,208.38 D47.C
29
  Top 0.5: D16.C 128.25,207.12 115.38,194.25 111.1,194.25 X2.9
30
  Bottom 0.5: 135.75,205.75 128.38,205.75 115.5,192.88 X2.28
  Bottom 0.506: 135.75,205.75 155.31,205.75 D48.C
31
  Top 0.5: D17.C 128.62,204.5 115.62,191.5 X2.10
32
  Bottom 0.5: 135.88,203.25 128.5,203.25 115.38,190.12 X2.29
  Bottom 0.506: 135.88,203.25 155.56,203.25 D49.C
33
  Top 0.5: X4.3 116.08,138.83 131.5,154.25 142.94,154.25 D18.C
34
  Bottom 0.5: 136.62,152.88 131.12,152.88 116,137.75 114.74,137.75 X4.22
  Bottom 0.506: 136.62,152.88 155.94,152.88 D50.C
35
  Top 0.5: X4.4 116.19,136.06 131.75,151.62 143.06,151.62 D19.C
  Top 0.506: 142.25,151.38 143.06,151.38 D19.C
36
  Bottom 0.5: 136.38,150.25 131.38,150.25 115.75,134.62 114.49,134.62 X4.23
  Bottom 0.506: 136.38,150.25 155.94,150.25 D51.C
37
  Top 0.5: X4.5 115.54,133.29 131.25,149 142.5,149
  Top 0.506: 142.5,149 143.19,149 D20.C
38
  Bottom 0.5: 136.5,147.62 131.12,147.62 115.62,132.12 114.63,132.12 X4.24
  Bottom 0.506: 136.5,147.62 155.94,147.62 D52.C
39
  Top 0.5: X4.6 115.42,130.55 131.25,146.38 142.75,146.38 142.88,146.25
  Top 0.506: D21.C 142.88,146.25 142.62,146.25
40
  Bottom 0.5: 136.62,144.88 131.25,144.88 115.62,129.25 114.52,129.25 X4.25
  Bottom 0.506: 136.62,144.88 156.06,144.88 D53.C
41
  Top 0.5: X4.7 115.41,127.78 131.12,143.5 D22.C
42
  Bottom 0.5: 137.25,142.12 130.75,142.12 115.25,126.62 114.64,126.62 X4.26
  Bottom 0.506: 137.25,142.12 156.06,142.12 D54.C
43
  Top 0.5: X4.8 115.26,125.01 131.12,140.88 D23.C
44
  Bottom 0.5: 137.5,139.62 131.38,139.62 115.38,123.62 114.44,123.62 X4.27
  Bottom 0.506: 137.5,139.62 156.19,139.62 D55.C
45
  Top 0.5: X4.9 115.77,122.27 131.62,138.12 D24.C
46
  Bottom 0.5: 137,136.88 131,136.88 115.12,121 114.55,121 X4.28
  Bottom 0.506: 137,136.88 156.19,136.88 D56.C
47
  Top 0.5: D25.C 131.5,135.5 115.5,119.5 X4.10
48
  Bottom 0.5: 136.5,134.25 131.25,134.25 115,118 114.55,118 X4.29
  Bottom 0.506: 136.5,134.25 156.19,134.25 D57.C
49
  Top 0.5: X5.3 116.33,64.33 131.88,79.88 D26.C
50
  Bottom 0.5: 137,78.62 132,78.62 116.5,63.12 115.11,63.12 X5.22
  Bottom 0.506: 137,78.62 156.44,78.62 D58.C
51
  Top 0.5: X5.4 116.69,61.56 132.38,77.25 D27.C
52
  Bottom 0.5: 137.5,76 131.62,76 116.12,60.5 115.23,60.5 X5.23
  Bottom 0.506: 137.5,76 156.44,76 D59.C
53
  Top 0.5: X5.5 115.79,58.79 131.88,74.88 143.94,74.88 D28.C
54
  Bottom 0.5: 137.12,73.5 132,73.5 116,57.5 115,57.5 X5.24
  Bottom 0.506: 137.12,73.5 156.44,73.5 D60.C
55
  Top 0.5: X5.6 115.8,56.05 132,72.25 143.81,72.25 D29.C
56
  Bottom 0.5: 137.75,70.88 131.38,70.88 115.88,55.38 115.64,55.38 X5.25
  Bottom 0.506: 137.75,70.88 156.69,70.88 D61.C
57
  Top 0.5: X5.7 116.28,53.28 132.25,69.25 143.38,69.25 143.5,69.12 143.69,69.12 D30.C
58
  Bottom 0.5: 137.62,68.12 131.5,68.12 115.5,52.12 115.14,52.12 X5.26
  Bottom 0.506: 137.62,68.12 156.56,68.12 D62.C
59
  Top 0.5: X5.8 116.14,50.51 132.38,66.75 D31.C
60
  Bottom 0.5: 138.12,65.38 131.16,65.38 X5.27
  Bottom 0.506: 138.12,65.38 156.69,65.38 D63.C
61
  Top 0.5: X5.9 115.89,47.77 132.38,64.25 143.81,64.25 D32.C
62
  Bottom 0.5: 137.75,62.75 131.3,62.75 X5.28
  Bottom 0.506: 137.75,62.75 156.88,62.75 D64.C
63
  Top 0.5: X5.10 116.38,45 132.75,61.38 143.93,61.38 D33.C
64
  Bottom 0.5: 138.12,60 131.29,60 X5.29
  Bottom 0.506: 138.12,60 156.76,60 D65.C
+5V
  Top 0.51: C3.1 38.12,199.15 38.5,198.77
  Top 0.61: IC2.20 IC2.21 49.7,196 47,196 44.23,198.77 IC2.7 | C4.1 56.25,177.62 56.12,177.5 | C5.1 56.12,141.38 56.25,141.25 | C7.1 56,105.75 56.25,105.5
  Top 0.813: U9.24 74.61,138.89 72.25,141.25 56.25,141.25 50.5,141.25 | R80.1 127.33,286.3 123.75,289.88 99.88,289.88 81.5,271.5 26.94,271.5 26.32,272.12 | DIS1.2 DIS1.3
  Top 1.016: 29.62,216.75 29.62,242.5 18.95,253.17 DIS1.3 19,260.56 19,264.5 26.32,271.81 26.32,272.12 U16.OUT | 29.62,216.75 29.62,198.25 | IC2.7 38.5,198.77 30.14,198.77 29.62,198.25 | 29.62,198.25 29.62,189.5 42,177.12 | 42,141.12 42,113.62 50.12,105.5 56.25,105.5 70.17,105.5 U10.24 | 50.5,141.25 42.12,141.25 42,141.12 | 42,141.12 42,177.12 | U8.24 71.14,175.36 69,177.5 56.12,177.5 42.38,177.5 42,177.12 | U7.24 74.61,214.14 71.88,216.88 29.75,216.88 29.62,216.75
  Bottom 1.016: C1.+ 27.94,274.88 26.32,276.5 U16.OUT
A  (via drill 0.7)
  Top 0.5: v64.45,172.82 U8.23 | U9.23 v64.45,135.35
  Top 0.506: U10.23 64.41,99.16 v64.38,99.12
  Top 0.51: IC2.2 47.41,211.47 48.62,210.25 60.88,210.25 62.12,211.5 74.56,211.5 U7.23
  Bottom 0.5: 73.34,211.56 64.45,202.66 v64.45,172.82 v64.45,135.35
  Bottom 0.506: v64.38,99.12 64.38,135.28 v64.45,135.35
  Bottom 0.51: 73.34,211.56 U7.23
B  (via drill 0.7)
  Top 0.5: U8.22 v65.72,170.28 | U9.22 v65.72,132.81
  Top 0.506: U10.22 v65.63,96.62 v65.62,96.62
  Top 0.51: IC2.3 47.2,208.93 48.38,207.75 62,207.75 63.25,209 74.59,209 U7.22
  Bottom 0.5: 73.34,209.01 65.72,201.4 v65.72,170.28 65.72,164.88 | v65.72,132.81 v65.72,162.62
  Bottom 0.506: v65.72,162.62 65.72,164.88 | v65.62,96.62 65.62,132.72 v65.72,132.81
  Bottom 0.51: 73.34,209.01 U7.22
C  (via drill 0.7)
  Top 0.5: U8.21 v66.99,167.74 | U9.21 v66.99,130.28
  Top 0.506: U10.21 66.92,94.08 v66.88,94.12
  Top 0.51: IC2.4 46.98,206.39 48.25,205.12 63,205.12 64.38,206.5 74.58,206.5 U7.21
  Bottom 0.5: 72.7,206.47 66.99,200.76 v66.99,167.74 66.99,160.75 | v66.99,130.28 66.99,157.62 | 66.99,158.62 66.99,160
  Bottom 0.506: 66.99,160 66.99,160.75 | 66.99,157.62 66.99,158.62 | v66.88,94.12 66.88,130.16 v66.99,130.28
  Bottom 0.51: 72.7,206.47 U7.21
D  (via drill 0.7)
  Top 0.5: v68.26,127.73 U9.20
  Top 0.506: 74.56,165.25 U8.20 74.53,165.12 | U10.20 68.29,91.54 v68.25,91.5
  Top 0.51: IC2.5 47.15,203.85 48.38,202.62 63.75,202.62 65.12,204 74.55,204 U7.20
  Bottom 0.5: 72.07,203.94 68.26,200.12 68.26,165.2 | 68.26,165.2 v68.26,127.73 | U8.20 68.26,165.2
  Bottom 0.506: v68.25,91.5 v68.25,127.72 v68.26,127.73
  Bottom 0.51: 72.07,203.94 U7.20
GND  (via drill 0.7)
  Top 0.5: U8.19 70.16,162.66 v70.12,162.62 | U9.19 62.55,125.19 v62.5,125.25
  Top 0.51: 44.25,202.5 44,202.5 43.88,202.62 40.38,202.62 | C3.2 38.52,202.15 39,202.62 | IC2.22 53.1,198.77 54,197.88 54.15,197.88 C8.2
  Top 0.61: v69.5,155.25 v62.5,155.25 | IC2.22 47.98,198.77 44.25,202.5 | C4.2 56.25,183.88 58.38,186 59.22,186 U7.12 | C5.2 57.85,145.9 U8.12 | C7.2 59.31,109.9 U9.12
  Top 0.813: U7.19 67.27,201.4 66,200.12 v62.5,200.12 | 40.38,202.62 39,202.62 35.5,202.62 v35.25,202.88
  Top 1.016: v33.75,196.25 42.3,196.25 IC2.8
  Bottom 0.5: v70.12,162.62 70.12,155.88 v69.5,155.25 | 61.75,156.25 61.75,156 v62.5,155.25
  Bottom 0.813: 62.3,147.42 62.5,147.62 | 61.95,109.95 62.5,110.5 | U10.19 62.5,89
  Bottom 1.016: DIS1.5 24.04,255.59 35.25,244.38 v35.25,202.88 35.25,197.75 v33.75,196.25 | U7.12 62.09,186.16 62.5,185.75 | 62.3,147.42 U8.12 | 61.95,109.95 U9.12 | 60.01,73.76 U10.12 | C2.2 26.04,281.48 U16.GND 30.75,281.75 31.38,281.75 | C6.- 31.38,281.75 | 31.38,281.75 C1.-
  Bottom 1.27: 60.01,73.76 62.5,76.25 62.5,89 62.5,110.5 v62.5,125.25 62.5,147.62 v62.5,155.25 62.5,185.75 62.5,186.25 | 62.5,186.25 v62.5,200.12 | 62.41,186.16 62.5,186.25 | SW3.1 32.25,294.5 35,291.75 35,289 | 35,289 35,283 33.75,281.75 30.75,281.75 | 13.75,275 13,275 8.25,279.75 X1.3 6,279.75 4.75,281 4.75,284.58 X1.2 | 13.75,275 18.75,275 22.25,278.5 22.25,281.35 C2.2 | SW1.2 51.45,280.05 42.5,289 35,289 | DIS1.1 13.88,265.25 | 13.88,265.25 13.88,274.88 13.75,275 | DIS1.5 24.04,262.96 21.5,265.5 14.12,265.5 13.88,265.25
  pour Bottom (isolate 0.813): 1,307 173.5,307 173.5,1 1,1
L1
  Top 0.5: R3.2 90.64,254.14 96.12,259.62 110.47,259.62 X3.11
L2
  Top 0.5: R4.2 91.71,213.46 92.62,214.38 92.62,254.12 96.86,258.36 X3.30
L3
  Top 0.406: 93.03,210.92 R5.2
  Top 0.5: X3.12 98.36,256.99 94.12,252.75 94.12,212.02 93.03,210.92
L4
  Top 0.406: R6.2 93.03,208.38
  Top 0.5: X3.31 99.84,255.59 95.62,251.38 95.62,210.98 93.03,208.38
L5
  Top 0.406: R7.2 92.12,205.84 92.39,205.84
  Top 0.5: X3.13 100.09,254.22 96.88,251 96.88,210.59 92.12,205.84
L6
  Top 0.406: R8.2 91.44,203.3
  Top 0.5: X3.32 100.32,252.82 98,250.5 98,209.86 91.44,203.3
L7
  Top 0.406: R9.2 90.95,200.44 91.75,200.44 92.07,200.44
  Top 0.5: X3.14 100.7,251.45 99,249.75 99,207.69 91.75,200.44
L8
  Top 0.406: R10.2 91.12,198.22
  Top 0.5: 91.12,198.22 91.84,198.22 100.12,206.5 100.12,249.38 100.88,250.12 113.38,250.12 X3.33
L9
  Top 0.406: R11.2 91.12,195.68 91.34,195.46
  Top 0.5: X3.15 101.93,248.68 101.25,248 101.25,205.38 91.34,195.46
L10
  Top 0.406: R12.2 90.64,192.99
  Top 0.5: X3.34 103.31,247.31 102.25,246.25 102.25,204.12 91.25,193.12 90.65,193.12 R12.2
L11
  Top 0.406: R13.2 91.12,190.6
  Top 0.5: 103.5,244.12 103.5,203.12 91.25,190.88 90.91,190.88 R13.2
  Top 0.51: X3.16 105.31,245.94 103.5,244.12
L12
  Top 0.406: R14.2 91.75,188.06
  Top 0.5: X3.35 106.42,244.54 104.62,242.75 104.62,200.93 91.75,188.06
L13
  Bottom 0.5: X3.17 101.67,243.17 96.62,238.12 96.62,192.14 R15.2
L14
  Bottom 0.5: X3.36 102.55,241.8 98.12,237.38 98.12,190 91.88,183.75 90.25,183.75 90.12,183.62 90.63,183.62 R16.2
L15
  Bottom 0.5: X3.18 103.4,240.4 99.25,236.25 99.25,189 91.62,181.38 90.94,181.38 R17.2
L16
  Bottom 0.5: X3.37 103.53,239.03 100.62,236.12 100.62,187.62 91.88,178.88 90.98,178.88 R18.2
L17
  Top 0.61: R19.2 91.73,175.36 105.12,188.75 111.06,188.75 X2.11
L18
  Top 0.51: 105.62,187.38 113.91,187.38 X2.30
  Top 0.61: 105.62,187.38 95.75,177.5 95.75,177.25 91.62,173.12 90.94,173.12 R20.2
L19
  Top 0.61: X2.12 111.07,186 106,186 97,177 97,175.88 91.38,170.25 90.67,170.25 R21.2
L20
  Top 0.5: R22.2 90.64,167.89
  Top 0.51: 106.12,184.5 113.83,184.5 X2.31
  Top 0.61: 106.12,184.5 98.25,176.62 98.25,174.38 91.75,167.88 90.77,167.88 R22.2
L21
  Top 0.61: X2.13 110.98,183.12 106.88,183.12 99.62,175.88 99.62,172.62 92.25,165.25 90.69,165.25 R23.2
L22
  Top 0.51: 107.75,181.88 113.87,181.88 X2.32
  Top 0.61: 107.75,181.88 101,175.12 101,171.75 91.88,162.62 90.67,162.62 R24.2
L23
  Top 0.61: X2.14 111,180.38 108,180.38 102.25,174.62 102.25,170.75 91.75,160.25 90.77,160.25 R25.2
L24
  Top 0.51: 108.75,179 113.84,179 X2.33
  Top 0.61: 108.75,179 103.62,173.88 103.62,169.38 92,157.75 90.81,157.75 R26.2
L25
  Top 0.61: X2.15 111.01,177.75 109.25,177.75 105.12,173.62 105.12,168.62 91.75,155.25 90.85,155.25 R27.2
L26
  Top 0.51: 109.75,176.25 109.88,176.38 113.86,176.38 X2.34
  Top 0.61: 109.75,176.25 106.5,173 106.5,167.62 91.5,152.62 90.76,152.62 R28.2
L27
  Top 0.61: R29.2 91.5,149.96 108,166.46 108,171.86 X2.16
L28
  Top 0.61: X2.35 116.25,171.22 116.25,167.25 114.56,165.56 114.5,165.62 113.5,165.62 95.3,147.42 R30.2
L29
  Bottom 0.5: X2.17 107.92,172.17 102.88,167.12
  Bottom 0.51: 102.88,167.12 102.88,167 90.62,154.75 90.62,148.7 R31.2
L30
  Bottom 0.406: 103.88,166.88 103.88,166.75 92.38,155.25 92.38,146.39 91.5,145.51
  Bottom 0.5: R32.2 91.5,145.51 | X2.36 107.8,170.8 103.88,166.88
L31
  Bottom 0.406: X2.18 107.65,169.4 93.38,155.12 93.38,145 91.25,142.88 90.74,142.88 R33.2
L32
  Bottom 0.406: 105.62,166.12 94.25,154.75 94.25,142.88 92,140.62
  Bottom 0.5: 91.12,140.44 R34.2 90.83,140.62 92,140.62 | X2.37 107.53,168.03 105.62,166.12
L33
  Top 0.5: X4.11 105.38,122.93 105.38,125.38 91.58,139.16 R35.2
L34
  Top 0.5: X4.30 114.41,115.38 110.25,115.38 103.88,121.75 103.88,124.25 91.5,136.62 R36.2
L35
  Top 0.5: X4.12 111.46,113.88 110,113.88 102.38,121.5 102.38,123.38 91.75,134 90.72,134 R37.2
L36
  Top 0.5: X4.31 114.39,112.62 109.5,112.62 101.12,121 101.12,122.62 92.2,131.54 R38.2
L37
  Top 0.5: X4.13 111.55,111.25 109.62,111.25 91.87,129 R39.2
L38
  Top 0.5: X4.32 114.37,109.88 109.5,109.88 92.91,126.47 R40.2
L39
  Top 0.5: X4.14 111.5,108.38 109.62,108.38 94.08,123.92 R41.2
L40
  Top 0.5: X4.33 114.34,107 109.5,107 95.11,121.39 R42.2
L41
  Top 0.5: X4.15 111.51,105.75 109.38,105.75 96.28,118.84 R43.2
L42
  Top 0.5: 91.12,116.31 R44.2 90.71,116.38 96.88,116.38 108.94,104.31 X4.34
L43
  Top 0.5: R45.2 91.25,113.77 | 91.25,113.77 91.44,113.77 | X4.16 108.94,102.94 98.12,113.75 91.27,113.75 91.25,113.77
L44
  Top 0.5: R46.2 91.44,111.22 91.54,111.12 99,111.12 108.58,101.54 X4.35
L45
  Bottom 0.5: 90.64,110.42 R47.2 99.3,109.95 109.12,100.12 111.53,100.12 X4.17
L46
  Bottom 0.5: X4.36 108.83,98.8 100.12,107.5 90.72,107.5 R48.2
L47
  Bottom 0.5: R49.2 101.25,104.88 108.62,97.5 111.48,97.5 X4.18
L48
  Bottom 0.5: 91.12,102.33 R50.2 90.68,102.38 102.25,102.38 108.59,96.03 X4.37
L49
  Top 0.5: R51.2 92.92,100.45 105.12,88.25 105.12,47.62 110.62,42.12 111.97,42.12 X5.11
L50
  Top 0.5: X5.30 110.27,40.86 104.12,47 104.12,87 93,98.12 90.79,98.12 R52.2
L51
  Top 0.5: X5.12 111.94,39.62 109.38,39.62 103.12,45.88 103.12,84.75 92.25,95.62 R53.2
L52
  Top 0.5: X5.31 109.41,38.09 102.12,45.38 102.12,84 93.04,93.08 R54.2 90.75,93.12
L53
  Top 0.5: X5.13 111.86,36.5 109.12,36.5 101,44.62 101,81.12 91.58,90.54 R55.2
L54
  Top 0.5: X5.32 108.8,35.32 100,44.12 100,79.5 91.5,88 R56.2
L55
  Top 0.5: X5.14 112.03,34 108.88,34 99.12,43.75 99.12,78.25 91.91,85.46 R57.2
L56
  Top 0.5: X5.33 109.05,32.58 98.25,43.38 98.25,76.38 91.62,83 90.78,83 R58.2
L57
  Top 0.5: X5.15 112.02,31.12 109.12,31.12 97.38,42.88 97.38,75.38 92.37,80.38 R59.2
L58
  Top 0.5: X5.34 109.06,29.81 96.38,42.5 96.38,74.38 92.88,77.88 90.74,77.88 R60.2
L59
  Top 0.5: R61.2 92.82,75.3 95.5,72.62 95.5,42 109,28.5 112.02,28.5 X5.16
L60
  Top 0.5: R62.2 92.49,73.01 94.62,70.88 94.62,41.5 109.12,27 114.88,27 X5.35
L61
  Bottom 0.5: R63.2 94.38,76.62 107.75,63.25 107.75,28.5 110.75,25.5 111.91,25.5 X5.17
L62
  Bottom 0.5: X5.36 110.08,24.3 106.38,28 106.38,63.25 95.5,74.12 91,74.12 R64.2
L63
  Bottom 0.5: X5.18 109.97,22.9 105.5,27.38 105.5,62.62 96.62,71.5 90.99,71.5 R65.2
L64
  Bottom 0.5: X5.37 109.84,21.53 104.5,26.88 104.5,62.25 97.62,69.12 91.08,69.12 R66.2
N$1
  Bottom 0.61: IC2.27 IC2.28
N$2
  Bottom 0.61: IC2.24 51.35,203.85 53,205.5 53,206 56,209 56,274.75 SW1.1
N$3
  Bottom 0.406: 38,262.38 38,258.88
  Bottom 0.61: DIS1.14 46.9,262.36 44.62,264.62 40.38,264.62 38,262.38 | 38,258.88 38.12,183.88 41.25,180.75 42.08,180.75 IC2.14
N$4
  Bottom 0.51: IC2.15 48,182.8 48,184.12 47.88,184.25 47.88,215.62 44.25,219.25
  Bottom 0.61: DIS1.13 44.35,259.25 | 44.35,259.25 44.35,258.02 | 44.25,219.25 44.25,259.14 44.35,259.25
N$5  (via drill 0.7)
  Top 0.51: v46.75,183.5 49.91,183.5 IC2.16
  Bottom 0.51: DIS1.12 41.81,219.31 46.88,214.25 46.88,183.62 v46.75,183.5
N$6  (via drill 0.7)
  Top 0.51: IC2.17 45.8,186.07 v45.75,186.12
  Bottom 0.51: v45.75,186.12 45.75,186.38 46,186.62 46,213.5 44.5,215
  Bottom 0.61: DIS1.11 39.27,220.22 44.5,215
N$7
  Top 0.506: R4.1 79.21,213.46 78.62,212.88 60.69,212.88 U7.2
N$8
  Top 0.506: R5.1 79.3,210.92 78.62,210.25 62.62,210.25 61.5,209.12 59.48,209.12 U7.3
N$9
  Top 0.506: R6.1 77.88,208.38 77.25,207.75 63.88,207.75 62.62,206.5 59.4,206.5 U7.4
N$10
  Top 0.506: R7.1 77.22,205.84 76.62,205.25 64.62,205.25 63.38,204 59.44,204 U7.5
N$11
  Top 0.506: R8.1 76.92,203.3 76.38,202.75 76.25,202.75 76.12,202.62 66.12,202.62 64.75,201.25 59.52,201.25 U7.6
N$12
  Top 0.5: 61.25,198.88 70.62,198.88 71.88,200.12
  Top 0.506: R9.1 77.14,200.76 76.5,200.12 71.88,200.12 | 61.25,198.88 59.39,198.88 U7.7
N$13
  Top 0.5: 62.38,196.38 71.75,196.38 72.88,197.5
  Top 0.506: R10.1 77.34,198.22 76.62,197.5 72.88,197.5 | U7.8 59.43,196.38 62.38,196.38
N$14
  Top 0.506: R11.1 77.68,195.68 77,195 62.12,195 61,193.88 59.47,193.88 U7.9
N$15
  Top 0.506: R12.1 77.39,193.14 76.75,192.5 62.12,192.5 60.88,191.25 59.38,191.25 U7.10
N$16
  Top 0.506: R13.1 77.47,190.6 76.88,190 61.62,190 60.5,188.88 59.55,188.88 U7.11
N$17
  Top 0.5: R14.1 80.33,188.06 78.42,186.16 U7.13
N$18
  Bottom 0.5: R15.1 81.59,186.16 79.06,188.69 U7.14
N$19
  Bottom 0.5: R16.1 73.34,183.62 72.07,184.88 72.07,189.33 73.97,191.24 U7.15
N$20
  Bottom 0.5: R17.1 73.34,181.07 70.8,183.62 70.8,191.24 73.34,193.78 U7.16
N$21
  Bottom 0.5: R18.1 73.97,178.53 69.53,182.98 69.53,193.78 72.07,196.31 U7.17
N$22
  Top 0.5: R19.1 78.42,175.36 77.15,174.09
  Top 0.506: 77.15,174.09 64.78,174.09 63.62,175.25 59.48,175.25 U8.1
N$23
  Top 0.5: R20.1 79.06,172.82 77.78,171.55 62.55,171.55 61.27,172.82 U8.2
N$24
  Top 0.5: R21.1 80.96,170.28 79.69,169.01 61.27,169.01 60.01,170.28 U8.3
N$25
  Top 0.5: R22.1 78.42,167.74 77.15,166.47
  Top 0.506: U8.4 65,167.75 66.25,166.5 77.12,166.5 77.15,166.47
N$26
  Top 0.5: R23.1 78.42,165.2 77.15,163.93
  Top 0.506: 77.15,163.93 64.82,163.93 63.5,165.25 59.42,165.25 U8.5
N$27
  Top 0.5: R24.1 78.42,162.66 77.15,161.39
  Top 0.506: 77.15,161.39 63.73,161.39 62.5,162.62 59.41,162.62 U8.6
N$28
  Top 0.5: R25.1 77.78,160.12 76.52,158.85
  Top 0.506: U8.7 61.38,160.12 62.62,158.88 76.49,158.88 76.52,158.85
N$29
  Top 0.5: R26.1 78.42,157.58 77.15,156.31 60.64,156.31 U8.8
N$30
  Top 0.5: R27.1 79.69,155.04 78.42,153.77 60.64,153.77 U8.9
N$31
  Top 0.5: R28.1 80.33,152.5 79.06,151.23 60.64,151.23 U8.10
N$32
  Top 0.5: R29.1 80.96,149.96 79.69,148.69 60.64,148.69 U8.11
N$33
  Top 0.5: R30.1 U8.13
N$34
  Bottom 0.5: R31.1 75.88,148.69 U8.14
N$35
  Bottom 0.5: R32.1 73.34,145.51 72.07,146.78 72.07,151.23 73.34,152.5 U8.15
N$36
  Bottom 0.5: R33.1 73.97,142.97 70.8,146.15 70.8,151.87 73.97,155.04 U8.16
N$37
  Bottom 0.5: R34.1 74.61,140.44 69.53,145.51 69.53,153.77 73.34,157.58 U8.17
N$38
  Top 0.5: R35.1 79.42,139.16 76.88,136.62 72.5,136.62 71.25,137.88 59.39,137.88 U9.1
N$39
  Top 0.5: R36.1 79.5,136.62 77,134.12 63,134.12 61.75,135.38 59.39,135.38 U9.2
N$40
  Top 0.5: R37.1 78.96,134.09 76.38,131.5 62.38,131.5 61,132.88 59.43,132.88 U9.3
N$41
  Top 0.5: R38.1 79.3,131.54 76.75,129 65.75,129 64.5,130.25 59.4,130.25 U9.4
N$42
  Top 0.5: R39.1 79.75,129 77.25,126.5 66.25,126.5 65,127.75 59.38,127.75 U9.5
N$43
  Top 0.5: R40.1 78.97,126.47 76.38,123.88
  Top 0.51: U9.6 60.68,125.19 62,123.88 76.38,123.88
N$44
  Top 0.5: R41.1 85.17,123.92 82.62,121.38 60.65,121.38 U9.7
N$45
  Top 0.5: R42.1 86.39,121.39 83.88,118.88 60.61,118.88 U9.8
N$46
  Top 0.5: R43.1 86.34,118.84 83.88,116.38 60.57,116.38 U9.9
N$47
  Top 0.5: R44.1 86.06,116.31 83.5,113.75 60.66,113.75 U9.10
N$48
  Top 0.5: R45.1 85.64,113.77 83.12,111.25 62.38,111.25 61.25,112.38 59.49,112.38 U9.11
N$49
  Top 0.5: U9.13 83.83,109.95 85.25,111.38 87.64,111.38 R46.1
N$50
  Bottom 0.506: R47.1 80.42,109.95 77.88,112.5 U9.14
N$51
  Bottom 0.506: R48.1 73.08,107.42 71.88,108.62 71.88,113.62 73.12,114.88 74.45,114.88 U9.15
N$52
  Bottom 0.506: R49.1 74,104.88 70.88,108 70.88,114.88 73.5,117.5 74.53,117.5 U9.16
N$53
  Bottom 0.506: R50.1 86.17,102.33 84.75,103.75 73.5,103.75 69.75,107.5 69.75,117.25 72.62,120.12 74.6,120.12 U9.17
N$54
  Top 0.5: 81.88,100.38 87.25,100.38 87.38,100.5 87.94,100.5 R51.1
  Top 0.51: 81.88,100.38 60.06,100.38 U10.1
N$55
  Top 0.5: 81.62,97.88 87.7,97.88 R52.1
  Top 0.51: 81.62,97.88 60.5,97.88 59.38,99 58.9,99 U10.2
N$56
  Top 0.5: 81.25,95.38 87.61,95.38 R53.1
  Top 0.51: 81.25,95.38 59.98,95.38 U10.3
N$57
  Top 0.5: 81.38,92.88 87.65,92.88 R54.1
  Top 0.51: 81.38,92.88 59.94,92.88 U10.4
N$58
  Top 0.5: 81.62,90.25 87.57,90.25 R55.1
  Top 0.51: U10.5 66.46,91.54 67.62,90.38 81.5,90.38 81.62,90.25
N$59
  Top 0.5: 81,87.75 87.61,87.75 R56.1
  Top 0.51: U10.6 71.12,89 72.38,87.75 81,87.75
N$60
  Top 0.5: 81.25,85.25 87.65,85.25 R57.1
  Top 0.51: 81.25,85.25 69.88,85.25 68.67,86.46 U10.7
N$61
  Top 0.5: 79.75,82.62 87.56,82.62 R58.1
  Top 0.506: 58.81,84 U10.8
  Top 0.51: 79.75,82.62 60.03,82.62 U10.8
N$62
  Top 0.5: 79.12,80.12 87.6,80.12 R59.1
  Top 0.51: 79.12,80.12 59.99,80.12 U10.9
N$63
  Top 0.5: 79.12,77.5 87.52,77.5 R60.1
  Top 0.506: 58.77,78.88 U10.10
  Top 0.51: 79.12,77.5 60.08,77.5 U10.10
N$64
  Top 0.5: 78.38,75 87.56,75 R61.1
  Top 0.51: 78.38,75 60.03,75 U10.11
N$65
  Top 0.5: 86.12,72.88 87.72,72.88 R62.1
  Top 0.506: 75.88,73.75 U10.13
  Top 0.51: 86.12,72.88 76.75,72.88 75.88,73.75
N$66
  Bottom 0.506: R63.1 74.29,76.62 U10.14
N$67
  Bottom 0.506: R64.1 87.45,74.08 84.5,71.12 72.5,71.12 70.88,72.75 70.88,77 72.5,78.62 73.76,78.62 U10.15
N$68
  Bottom 0.506: R65.1 87.41,71.54 86,70.12 72.25,70.12 69.88,72.5 69.88,78 73.25,81.38 U10.16
N$69  (via drill 0.7)
  Top 0.51: IC2.18 45.89,188.61 44.62,189.88 39.62,189.88
  Top 0.61: v36,189.88 39.62,189.88
  Bottom 0.61: DIS1.6 26.57,259.93 36.88,249.62 36.88,190.75 v36,189.88
N$70  (via drill 0.7)
  Top 0.51: v31.5,192.5 31.62,192.5 31.75,192.38 45.25,192.38 46.5,191.12 49.91,191.12 IC2.19
  Bottom 1.016: DIS1.4 21.5,254.38 31.38,244.5 31.38,192.62 v31.5,192.5
N$72  (via drill 0.7)
  Top 0.51: v85.62,216 R3.1
  Top 0.61: 87.67,215.88 R3.1
  Bottom 0.51: U7.1 71.47,214.09 73.38,216 v85.62,216
N$95
  Bottom 1.27: SW3.2 17,288.45 D68.A
N$109
  Top 0.51: C8.1 50.22,201.03 IC2.23 | D35.A 163.31,280.19 D34.A 163.45,283.05 | R80.2 163.45,283.45 163.25,283.25
  Top 0.813: D2.A D3.A 150.19,274.85 D4.A 150.32,272.01 D5.A D6.A 150.19,266.68 D7.A 150.07,264.07 D8.A | D17.A 150.56,204.62 D16.A 150.44,207.25 D15.A D14.A D13.A 150.31,215.25 D12.A D11.A 150.31,223 D10.A | 150.81,154.25 D18.A 150.69,151.62 D19.A 150.81,149 D20.A 150.94,146.38 D21.A 151.06,143.62 D22.A D23.A 151.19,138.25 D24.A D25.A | D26.A 151.56,77.36 D27.A 151.45,74.98 D28.A 151.69,72.25 D29.A D30.A 151.56,66.88 D31.A 151.69,64.25 D32.A 151.56,61.37 D33.A | D35.A D36.A 163.31,272 D37.A D38.A D39.A D40.A | D49.A 164.31,204.62 D48.A D47.A 164.19,209.88 D46.A 164.31,212.62 D45.A 164.06,215.38 D44.A D43.A D42.A | D51.A 164.94,151.38 D52.A 164.94,146.38 D53.A D54.A D55.A D56.A D57.A | D58.A 165.31,77.5 D59.A 165.44,74.88 D60.A 165.31,72.12 D61.A 165.31,71.88 D62.A 165.31,66.62 D63.A 165.44,63.97 D64.A 165.57,61.21 D65.A
  Top 1.016: D8.A 150.07,263.82 D9.A 149.94,260.84 149.94,223.62 D10.A | D41.A 163.69,263.62 D40.A | 150.81,154.25 150.81,157 | 150.81,157 150.81,201.12 | 150.81,201.12 150.81,204.12 D17.A | 150.81,157 150.94,156.88 160.5,156.88 163.25,154.12 D50.A D51.A | 164.31,204.62 164.31,202.31 163.25,201.25 150.94,201.25 150.81,201.12 | D28.A 151.69,83.12 | 151.69,83.12 151.69,135.12 D25.A | 151.69,83.12 152.06,82.75 162.75,82.75 165.06,80.44 165.06,80.12 D58.A | 163.45,283.05 163.25,283.25 153.02,283.25 D2.A
  Bottom 0.406: 101.25,244.62 109.62,244.62 109.75,244.5 111.62,244.5 111.75,244.62 111.75,244.88 112.75,245.88
  Bottom 0.51: 71.62,212.38 72.12,212.88 92.88,212.88 95.25,215.25
  Bottom 0.61: 150.14,280.38 D2.A | IC2.23 51.31,201.31 55.12,205.12 64.38,205.12 71.62,212.38 | 112.75,245.88 114.38,245.88 116,247.5 116,253.25 121,258.25 160.94,258.25 D41.A | 95.25,215.25 95.25,238.62 101.25,244.62
N$118
  Top 1.27: D68.C 16.88,279.88 21.29,284.29 U16.IN
  Bottom 0.813: C2.1 26.3,284.27 U16.IN 26.25,284.36 26.25,286 28.88,288.62 C6.+
N$119
  Bottom 1.27: X1.1 11.07,292.58 SW3.3
PD4
  Top 0.406: 47.25,197.5 51.75,197.5 53.12,196.12 56.25,196.12 57.75,197.62 61.5,197.62
  Top 0.51: IC2.6 43.44,201.31 47.25,197.5 | U7.18 74.59,198.88 72.38,198.88 71.12,197.62 61.5,197.62
PD5  (via drill 0.7)
  Top 0.51: U8.18 74.49,160 63.25,160 61.88,161.38 v47.62,161.38
  Bottom 0.406: 44.38,187.38 44.75,187 44.75,185.5 45.75,184.5 45.75,182.62 47.62,180.75 v47.62,161.38
  Bottom 0.51: IC2.11 43.14,188.61 44.38,187.38
PD6  (via drill 0.7)
  Top 0.406: U9.18 61.84,122.66 60.62,123.88 57.5,123.88 57,123.88 56.88,123.75
  Top 0.51: v46.62,123.88 57.5,123.88
  Bottom 0.406: IC2.12 42.8,186.07 45,183.88 45,181.5 46.5,180
  Bottom 0.51: 46.5,180 46.5,124 v46.62,123.88
PD7  (via drill 0.7)
  Top 0.51: U10.18 71.17,86.46 69.88,87.75 56.5,87.75 56.38,87.88 v45.12,87.88
  Bottom 0.406: IC2.13 42.84,183.53 44.25,182.12 44.25,180.5 45.12,179.62 v45.12,87.88
U10.17
  Bottom 0.506: R66.1 72,69 | 68.62,73.38 68.62,79.5
  Bottom 0.51: 72,69 71.62,69 68.62,72 68.62,73.38 | 68.62,79.5 68.62,80.17 72.38,83.92 U10.17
